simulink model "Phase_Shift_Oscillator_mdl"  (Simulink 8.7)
settings: Solver=ode23s  StartTime=0.0  StopTime=10.0  RelTol=1e-6  AbsTol=1e-6
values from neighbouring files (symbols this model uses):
  beta = 60    [Phase_Shift_Oscillator.m]
  C = 0.001    [Phase_Shift_Oscillator.m]
  Q30 = C*V30    (= 0.0001)    [Phase_Shift_Oscillator.m]
  R = 1    [Phase_Shift_Oscillator.m]
  tau = 0.000001    (= 1e-06)    [Phase_Shift_Oscillator.m]
  VM = 12    [Phase_Shift_Oscillator.m]

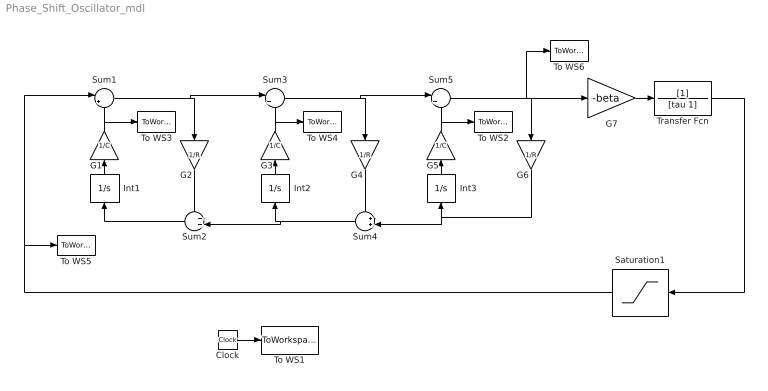
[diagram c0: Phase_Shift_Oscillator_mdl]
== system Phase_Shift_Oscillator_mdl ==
  Clock : Clock
  G1 : Gain  Gain=1/C
  G2 : Gain  Gain=1/R
  G3 : Gain  Gain=1/C
  G4 : Gain  Gain=1/R
  G5 : Gain  Gain=1/C
  G6 : Gain  Gain=1/R
  G7 : Gain  Gain=-beta
  Int1 : Integrator
  Int2 : Integrator
  Int3 : Integrator  InitialCondition=Q30
  Saturation1 : Saturate  UpperLimit=VM  LowerLimit=-VM
  Sum1 : Sum  Inputs=|+-
  Sum2 : Sum  Inputs=++|
  Sum3 : Sum  Inputs=|+-
  Sum4 : Sum  Inputs=++|
  Sum5 : Sum  Inputs=|+-
  To WS1 : ToWorkspace  VariableName=t  SampleTime=-1
  To WS2 : ToWorkspace  VariableName=V3  SampleTime=-1
  To WS3 : ToWorkspace  VariableName=V1  SampleTime=-1
  To WS4 : ToWorkspace  VariableName=V2  SampleTime=-1
  To WS5 : ToWorkspace  VariableName=V0  SampleTime=-1
  To WS6 : ToWorkspace  VariableName=Vp  SampleTime=-1
  Transfer Fcn : TransferFcn  Denominator=[tau 1]
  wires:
  Int1/1 -> G1/1
  G2/1 -> Sum2/1
  Sum2/1 -> Int1/1
  Sum1/1 -> G2/1, Sum3/1
  Int2/1 -> G3/1
  G4/1 -> Sum4/1
  Sum3/1 -> G4/1, Sum5/1
  Int3/1 -> G5/1
  Sum4/1 -> Int2/1, Sum2/2
  G6/1 -> Int3/1, Sum4/2
  Sum5/1 -> To WS6/1, G6/1, G7/1
  G7/1 -> Transfer Fcn/1
  Clock/1 -> To WS1/1
  G1/1 -> Sum1/2, To WS3/1
  G3/1 -> Sum3/2, To WS4/1
  G5/1 -> Sum5/2, To WS2/1
  Transfer Fcn/1 -> Saturation1/1
  Saturation1/1 -> Sum1/1, To WS5/1
